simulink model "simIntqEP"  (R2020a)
settings: Solver=ode15s  StartTime=0.0  StopTime=tsim  RelTol=1e-3

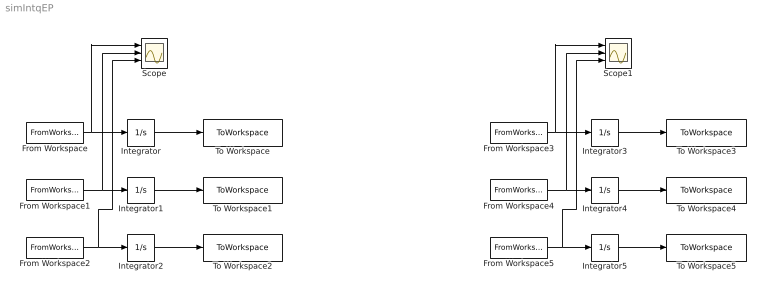
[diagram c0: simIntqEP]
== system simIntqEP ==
  From Workspace : FromWorkspace  VariableName=[tSRC qEPSRC]
  From Workspace1 : FromWorkspace  VariableName=[t3C qEP3C]
  From Workspace2 : FromWorkspace  VariableName=[tgrid qEPMPC]
  From Workspace3 : FromWorkspace  VariableName=[tSRC qDSRC]
  From Workspace4 : FromWorkspace  VariableName=[t3C qD3C]
  From Workspace5 : FromWorkspace  VariableName=[tgrid qDMPC]
  Integrator{,1..5} (6 alike) : Integrator
  Scope : Scope  NumInputPorts=3
  Scope1 : Scope  NumInputPorts=3
  To Workspace : ToWorkspace  VariableName=intSRC  SampleTime=-1
  To Workspace1 : ToWorkspace  VariableName=int3C  SampleTime=-1
  To Workspace2 : ToWorkspace  VariableName=intMPC  SampleTime=-1
  To Workspace3 : ToWorkspace  VariableName=intDSRC  SampleTime=-1
  To Workspace4 : ToWorkspace  VariableName=intD3C  SampleTime=-1
  To Workspace5 : ToWorkspace  VariableName=intDMPC  SampleTime=-1
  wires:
  From Workspace/1 -> Scope/1, Integrator/1
  From Workspace2/1 -> Scope/3, Integrator2/1
  From Workspace1/1 -> Scope/2, Integrator1/1
  Integrator/1 -> To Workspace/1
  Integrator2/1 -> To Workspace2/1
  Integrator1/1 -> To Workspace1/1
  From Workspace3/1 -> Scope1/1, Integrator3/1
  Integrator4/1 -> To Workspace4/1
  Integrator5/1 -> To Workspace5/1
  From Workspace4/1 -> Scope1/2, Integrator4/1
  From Workspace5/1 -> Scope1/3, Integrator5/1
  Integrator3/1 -> To Workspace3/1
